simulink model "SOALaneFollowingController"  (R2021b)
settings: Solver=FixedStepDiscrete  StartTime=0.0  StopTime=10.0  RelTol=1e-3

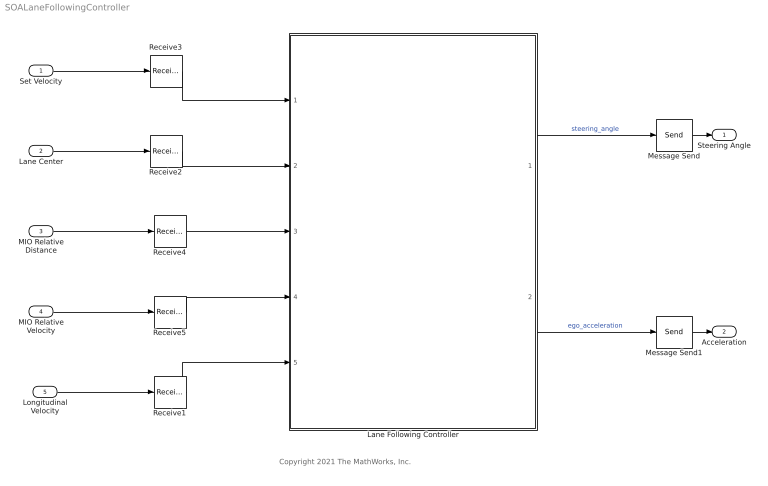
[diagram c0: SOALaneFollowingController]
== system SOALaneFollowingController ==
  note: Copyright 2021 The MathWorks, Inc.
  Set Velocity : Inport  OutputPortMessageModes=m  Unit=m/s
  Lane Center : Inport  OutputPortMessageModes=m  Port=2  OutDataTypeStr=Bus: BusLaneCenter
  MIO Relative Distance : Inport  OutputPortMessageModes=m  Port=3
  MIO Relative Velocity : Inport  OutputPortMessageModes=m  Port=4
  Longitudinal Velocity : Inport  OutputPortMessageModes=m  Port=5  Unit=m/s
  Lane Following Controller : ModelReference  ModelNameDialog=LaneFollowingController  SimulationMode=Normal  ModelReferenceVersion=4.4
  Message Send : Send  OutputPortMessageModes=m
  Message Send1 : Send  OutputPortMessageModes=m
  Receive1 : Receive  InputPortMessageModes=m  UseInternalQueue=off  QueueOverwriting=on  QueueLength=1  QueueType=LIFO  InitialValue=egoVehDyn.VLong0
  Receive2 : Receive  InputPortMessageModes=m  UseInternalQueue=off  QueueOverwriting=on  QueueLength=1  QueueType=LIFO
  Receive3 : Receive  InputPortMessageModes=m  UseInternalQueue=off  QueueOverwriting=on  QueueLength=1  QueueType=LIFO  InitialValue=v_set
  Receive4 : Receive  InputPortMessageModes=m  UseInternalQueue=off  QueueOverwriting=on  QueueLength=1  QueueType=LIFO
  Receive5 : Receive  InputPortMessageModes=m  UseInternalQueue=off  QueueOverwriting=on  QueueLength=1  QueueType=LIFO
  Steering Angle : Outport  InputPortMessageModes=m  Unit=rad  PortDimensions=1  VectorParamsAs1DForOutWhenUnconnected=off
  Acceleration : Outport  InputPortMessageModes=m  Port=2  Unit=m/s^2  PortDimensions=1  VectorParamsAs1DForOutWhenUnconnected=off
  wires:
  Lane Following Controller/1 -> Message Send/1  "steering_angle"
  Receive3/1 -> Lane Following Controller/1
  Set Velocity/1 -> Receive3/1
  Lane Following Controller/2 -> Message Send1/1  "ego_acceleration"
  Receive1/1 -> Lane Following Controller/5
  Longitudinal Velocity/1 -> Receive1/1
  Receive5/1 -> Lane Following Controller/4
  MIO Relative Velocity/1 -> Receive5/1
  Receive2/1 -> Lane Following Controller/2
  Lane Center/1 -> Receive2/1
  Receive4/1 -> Lane Following Controller/3
  MIO Relative Distance/1 -> Receive4/1
  Message Send/1 -> Steering Angle/1
  Message Send1/1 -> Acceleration/1
